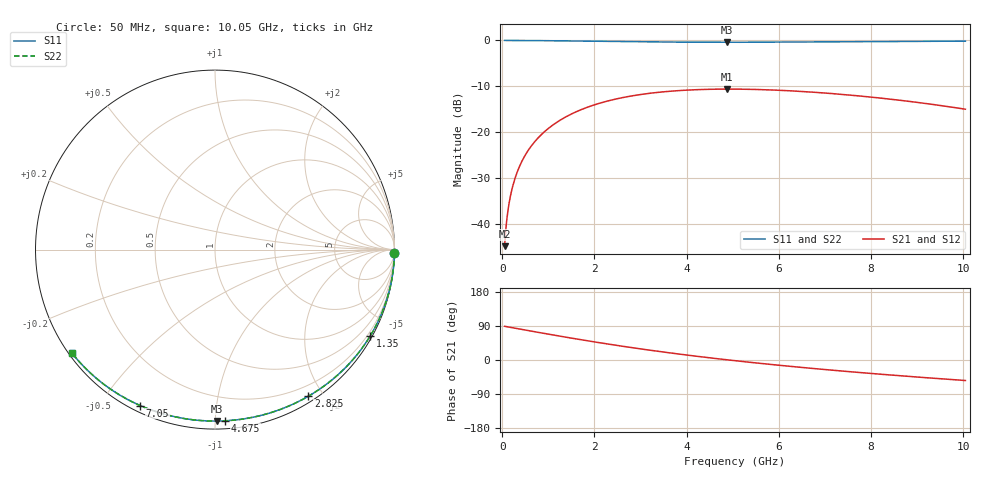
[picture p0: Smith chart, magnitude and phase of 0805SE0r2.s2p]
! AVX Thin Film Operation		Date: August 2001
! Description: Accu-P® Series, Thin Film, SMD, RF Capacitor
! Part Number: 08051J0R2ABT
! 50 MHz  -  10.05 GHz
! Serial Measurements
# mhz S db R 50
!	S11		S21		S12		S22
!	dB	Phase	dB	Phase	dB	Phase	dB	Phase
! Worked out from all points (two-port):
!   401 points, 50 MHz to 10.05 GHz, reference 50 ohm
!   highest |S21| = -10.62 dB at 4.875 GHz (marker M1); lowest = -44.9 dB at 50 MHz (marker M2)
!   |S21| within 3 dB of the highest: 2.141 GHz to 9.08 GHz (6.938 GHz wide, 124 % of centre)
!   lowest |S11| = -0.4 dB at 4.875 GHz (marker M3), VSWR 43.88, Z = 2.3 - j50.5 ohm
!   |S11| at or under -10 dB: nowhere
!   |S22| runs from -0.4 to 0.0 dB; largest |S21 - S12| = 0
!   S11 on the Smith chart (normalised r, x): 50 MHz: open; 1.35 GHz: 0.08, -3.84; 2.825 GHz: 0.07, -1.82; 4.675 GHz: 0.05, -1.06; 7.05 GHz: 0.03, -0.63; 10.05 GHz: 0.01, -0.32
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50  -0.00 -1.1  -44.93 89.0  -44.93 89.0  -0.00 -1.1
75  -0.00 -1.7  -41.41 88.4  -41.41 88.4  -0.00 -1.7
150  -0.00 -3.3  -35.39 86.7  -35.39 86.7  -0.00 -3.3
200  -0.00 -4.4  -32.90 85.6  -32.90 85.6  -0.00 -4.4
300  -0.01 -6.6  -29.39 83.4  -29.39 83.4  -0.01 -6.6
425  -0.01 -9.3  -26.39 80.7  -26.39 80.7  -0.01 -9.4
600  -0.02 -13.2  -23.45 76.8  -23.45 76.8  -0.02 -13.2
800  -0.03 -17.5  -21.04 72.5  -21.04 72.5  -0.03 -17.5
1050  -0.06 -22.9  -18.82 67.1  -18.82 67.1  -0.06 -22.9
1350  -0.09 -29.2  -16.85 60.8  -16.85 60.8  -0.09 -29.2
1725  -0.14 -36.8  -15.06 53.2  -15.06 53.2  -0.14 -36.8
2275  -0.21 -47.5  -13.25 42.5  -13.25 42.5  -0.21 -47.6
2825  -0.28 -57.6  -12.09 32.4  -12.09 32.4  -0.28 -57.6
3400  -0.34 -67.4  -11.31 22.6  -11.31 22.6  -0.34 -67.4
4025  -0.38 -77.2  -10.84 12.7  -10.84 12.7  -0.38 -77.3
4675  -0.39 -86.7  -10.64 3.3  -10.64 3.3  -0.39 -86.7
4875  -0.40 -89.4  -10.62 0.5  -10.62 0.5  -0.40 -89.5
5050  -0.40 -91.8  -10.63 -1.8  -10.63 -1.8  -0.40 -91.8
6725  -0.34 -112.1  -11.29 -22.2  -11.29 -22.2  -0.34 -112.2
7050  -0.32 -115.6  -11.52 -25.7  -11.52 -25.7  -0.32 -115.7
8400  -0.24 -129.3  -12.80 -39.4  -12.80 -39.4  -0.24 -129.3
10050  -0.14 -144.0  -15.02 -54.1  -15.02 -54.1  -0.14 -144.1
